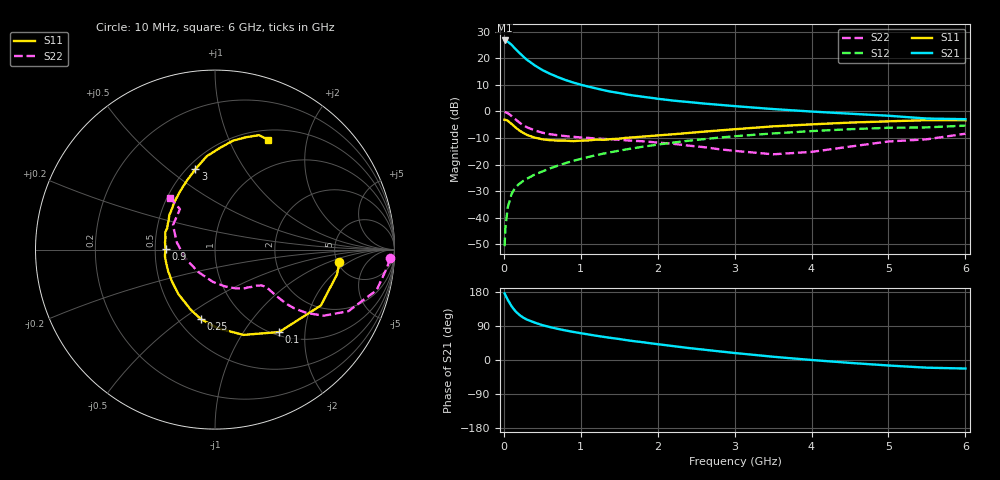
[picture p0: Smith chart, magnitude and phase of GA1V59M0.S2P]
! Infineon Technologies  Discrete & RF Semiconductors
! BF775
! Si NPN RF Bipolar Junction Transistor in SOT23
! VCE = 1.5 V  IC = 9 mA
! Common Emitter S-Parameters:  May  1996
# GHz  S  MA  R  50
!  f  S11  S21  S12  S22
! GHz  MAG  ANG  MAG  ANG  MAG  ANG  MAG  ANG
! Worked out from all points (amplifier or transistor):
!   36 points, 10 MHz to 6 GHz, reference 50 ohm
!   highest |S21| = 26.7 dB at 10 MHz (marker M1)
!   |S21| within 3 dB of that: start of sweep to 144.1 MHz
!   unconditionally stable (mu >= 1): 535.2 MHz to 4.216 GHz; 5.254 GHz to end of sweep
!   at 250 MHz: K = 0.68, MSG = 23.5 dB, |S12| = -26.2 dB
!   at 1.4 GHz: K = 1.15, MAG = 9.0 dB, |S12| = -15.3 dB
!   at 6 GHz: K = 1.00, MAG = 1.2 dB, |S12| = -5.4 dB
!   S11 on the Smith chart (normalised r, x): 10 MHz: 5.19, -1.42; 100 MHz: 1.06, -1.47; 250 MHz: 0.64, -0.59; 900 MHz: 0.57, +0.00; 3 GHz: 0.55, +0.63; 6 GHz: 0.62, +1.41
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0.01  0.6967 -5.8  21.65 175.7  0.0029 83.7  0.9772 -2.8
0.02  0.6938 -11.5  21.28 171.2  0.0063 81.4  0.9646 -5.8
0.05  0.6671 -27.8  20.57 159.3  0.0154 76.7  0.9284 -14.1
0.1  0.5819 -52.1  17.95 142.1  0.0279 67.7  0.8186 -24.8
0.15  0.5011 -71.5  15.01 128.8  0.037 62.0  0.7089 -31.3
0.2  0.4391 -87.7  12.74 119.5  0.0432 59.4  0.6198 -34.7
0.25  0.3958 -101.3  10.85 112.1  0.0489 58.6  0.5505 -36.5
0.3  0.3613 -111.9  9.374 106.7  0.0541 58.4  0.5032 -37.2
0.4  0.3211 -129.4  7.378 98.8  0.0645 59.2  0.4388 -37.1
0.5  0.2981 -143.5  6.011 92.0  0.0739 60.1  0.3968 -36.7
0.6  0.2873 -155.4  5.104 86.9  0.0843 61.1  0.372 -36.4
0.7  0.2821 -164.6  4.43 82.2  0.095 61.5  0.3554 -36.5
0.9  0.2757 179.4  3.5 74.2  0.117 61.4  0.3318 -37.3
1.1  0.2837 166.8  2.924 67.4  0.1389 60.8  0.3163 -39.4
1.3  0.2918 155.9  2.503 61.0  0.1608 59.7  0.3026 -41.9
1.6  0.3188 143.1  2.082 52.2  0.1934 56.9  0.2847 -47.3
2.2  0.3704 123.2  1.597 36.7  0.2584 50.5  0.2455 -61.8
3  0.4612 103.7  1.257 18.5  0.3404 40.2  0.1806 -93.6
3.5  0.5225 95.0  1.106 8.6  0.3847 33.3  0.1556 -126.5
4.5  0.6152 80.6  0.905 -7.6  0.4622 19.7  0.2172 169.1
5.5  0.6834 68.9  0.733 -20.3  0.4998 5.6  0.2983 130.9
6  0.6794 64.1  0.713 -22.5  0.5398 1.6  0.3796 130.9
